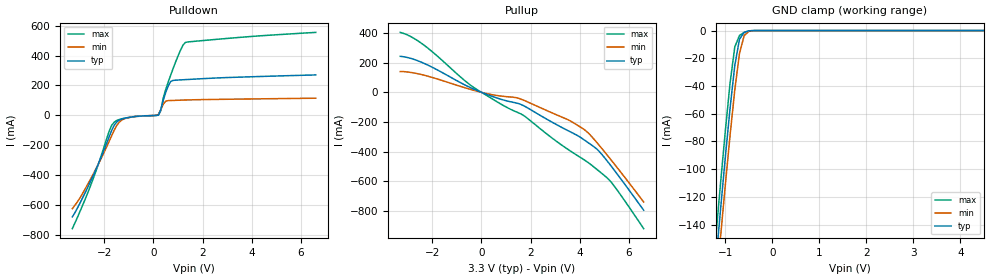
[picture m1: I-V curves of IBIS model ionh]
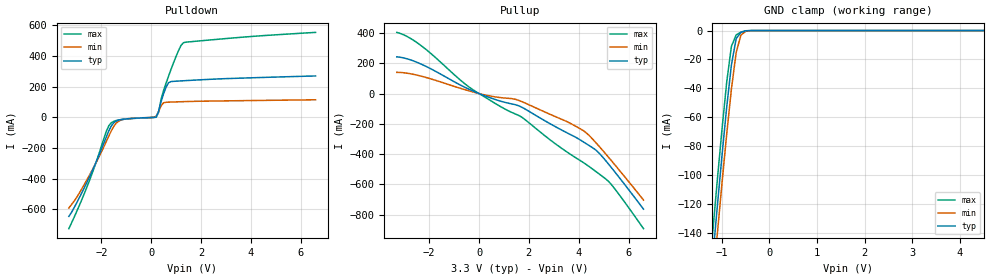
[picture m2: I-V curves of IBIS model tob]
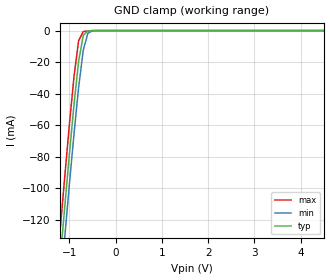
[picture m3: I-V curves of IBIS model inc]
[IBIS Ver]   2.1
[File name]   18512.ibs
[File Rev]   1.0   | from silicon model only
[Date]   97215
[Source]   Silicon-level SPICE model at Texas Instruments (ALEY)
[Notes]
   3.3-V ABT SCAN TEST DEVICES WITH 18-BIT UNIVERSAL BUS TRANSCEIVERS
   Release 1.0) 97215 ALEY - initial release
   includes all available commercial packages:
   DGG=64TSSOP (no-coupling model)
[Disclaimer]
   Property of Texas Instruments Incorporated.  Unauthorized
   reproduction and/or distribution is strictly prohibited.
   This product is protected under copyright law.
   Created 1997, (C) Copyright 1997, Texas Instruments Incorporated.
   All Rights Reserved
   UNLESS THERE IS A SIGNED, WRITTEN AGREEMENT TO THE
   CONTRARY, TEXAS INSTRUMENTS ("TI") IS PROVIDING THE IBIS
   MODELS "AS IS" AND WITHOUT ANY WARRANTY, EXPRESSED OR
   IMPLIED.  TI assumes no liability for:
   1) the accuracy of the IBIS models provided to your
   company;
   2) the proper functioning of these IBIS models in your
   design or for any resulting applications; or
   3) infringement of patents, copyrights or intellectual
   property rights resulting from your use of these IBIS
   models.
   TI provides IBIS Models as a service to our customers.
   You and your company shall not distribute, sell or give
   these models to anyone else without prior written
   permission from TI.
   TI reserves the right to make changes to our products or
   to discontinue any semiconductor product or service
   without notice, and advises our customers to obtain the
   latest version of relevant information to verify, before
   placing orders, that the information being relied on is
   current.
   Please be aware that your receipt and use of the IBIS
   information provided shall serve as acceptance of these
   terms and conditions.  If you do not accept these terms,
   you should return or destroy the IBIS models and any
   other accompanying information immediately.
[Component]   SN74LVT18512DGG
[Manufacturer]  Texas Instruments
[Package]
| 64-pin TSSOP (suffix = DGG)
| variable   typ   min   max
R_pkg   50m   NA   NA
L_pkg   4.0n   NA   NA
C_pkg   0.5p   NA   NA
[Pin]   signal_name   model_name   R_pin   L_pin   C_pin
1   1CLKAB   inc   0.057   5.49n   0.82p
2   1LEAB   inc   0.058   5.10n   0.90p
3   1OEAB#   inu   0.062   4.79n   0.80p
4   1A1   ionh   0.057   4.41n   0.72p
5   1A2   ionh   0.056   4.09n   0.66p
6   GND   GND   0.058   3.86n   0.57p
7   1A3   ionh   0.052   3.54n   0.54p
8   1A4   ionh   0.050   3.34n   0.50p
9   1A5   ionh   0.048   3.12n   0.40p
10   Vcc   POWER   0.046   3.02n   0.39p
11   1A6   ionh   0.049   2.86n   0.35p
12   1A7   ionh   0.046   2.73n   0.34p
13   1A8   ionh   0.043   2.62n   0.33p
14   GND   GND   0.043   2.53n   0.31p
15   1A9   ionh   0.046   2.58n   0.30p
16   2A1   ionh   0.045   2.56n   0.24p
17   2A2   ionh   0.045   2.56n   0.24p
18   2A3   ionh   0.046   2.58n   0.30p
19   GND   GND   0.043   2.53n   0.31p
20   2A4   ionh   0.043   2.62n   0.33p
21   2A5   ionh   0.046   2.73n   0.34p
22   2A6   ionh   0.049   2.86n   0.35p
23   Vcc   POWER   0.046   3.02n   0.39p
24   2A7   ionh   0.048   3.12n   0.40p
25   2A8   ionh   0.050   3.34n   0.50p
26   2A9   ionh   0.052   3.54n   0.54p
27   GND   GND   0.058   3.86n   0.57p
28   2OEAB#   inu   0.056   4.09n   0.66p
29   2LEAB   inc   0.057   4.41n   0.72p
30   2CLKAB   inc   0.062   4.79n   0.80p
31   TDO   tob   0.058   5.10n   0.90p
32   TMS   inu   0.057   5.49n   0.82p
33   TCK   int   0.057   5.49n   0.82p
34   TDI   inu   0.058   5.10n   0.90p
35   2CLKBA   inc   0.062   4.79n   0.80p
36   2LEBA   inc   0.057   4.41n   0.72p
37   2OEBA#   inu   0.056   4.09n   0.66p
38   GND   GND   0.058   3.86n   0.57p
39   2B9   ionh   0.052   3.54n   0.54p
40   2B8   ionh   0.050   3.34n   0.50p
41   2B7   ionh   0.048   3.12n   0.40p
42   Vcc   POWER   0.046   3.02n   0.39p
43   2B6   ionh   0.049   2.86n   0.35p
44   2B5   ionh   0.046   2.73n   0.34p
45   2B4   ionh   0.043   2.62n   0.33p
46   GND   GND   0.043   2.53n   0.31p
47   2B3   ionh   0.046   2.58n   0.30p
48   2B2   ionh   0.045   2.56n   0.24p
49   2B1   ionh   0.045   2.56n   0.24p
50   1B9   ionh   0.046   2.58n   0.30p
51   GND   GND   0.043   2.53n   0.31p
52   1B8   ionh   0.043   2.62n   0.33p
53   1B7   ionh   0.046   2.73n   0.34p
54   1B6   ionh   0.049   2.86n   0.35p
55   Vcc   POWER   0.046   3.02n   0.39p
56   1B5   ionh   0.048   3.12n   0.40p
57   1B4   ionh   0.050   3.34n   0.50p
58   1B3   ionh   0.052   3.54n   0.54p
59   GND   GND   0.058   3.86n   0.57p
60   1B2   ionh   0.056   4.09n   0.66p
61   1B1   ionh   0.057   4.41n   0.72p
62   1OEBA#   inu   0.062   4.79n   0.80p
63   1LEBA   inc   0.058   5.10n   0.90p
64   1CLKBA   inc   0.057   5.49n   0.82p
| Models and submodels in the file (5): ionh (I/O), tob (3-state), inc (Input), int (Input), inu (Input)
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[Model]   ionh
| high-drive I/O buffer (NO bus-hold)
| ibuf.lvta (97212 ALEY)
| tob.lvta  (97212 ALEY)
| pad.lvta  (97212 ALEY)
| Signals   1A1..1A9, 2A1..2A9, 1B1..1B9, 2B1..2B9
Model_type  I/O
Polarity   Non-Inverting
Enable   Active-Low
Vinl = 0.8V
Vinh = 2.0V
| variable   typ   min   max
C_comp   10p   NA   NA
[Temperature Range]   50   100   0
[Voltage range]   3.3   3   3.6
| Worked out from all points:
|   slope of the pulldown table from 0 to 0.495 V, typ, clamps not added: 3.25 ohm
|   slope of the pullup table from 0 to 0.495 V, typ, clamps not added: 16.2 ohm
|   GND clamp passes 1 mA (typ) near -0.57 V on its own axis
|Process range|   weak   strong
[pullup]
|   50C:3.3V:   100C:3V:weak   0C:3.6V:strong
|   Voltage   I(typ)   I(min)   I(max)
-3.3V     242.7mA    140.2mA    404.2mA
-2.8V     225.4mA    132.2mA    369.3mA
-2.3V     192.9mA    114.1mA    313.8mA
-300mV    20.86mA    13.18mA    31.49mA
700mV     -41.88mA   -23.15mA   -70.19mA
1.5V      -75.36mA   -39.76mA   -137.7mA
1.8V      -97.58mA   -58.88mA   -166.1mA
3.6V      -265.1mA   -191.5mA   -393.7mA
4.3V      -334.7mA   -267.1mA   -468.9mA
4.7V      -383.4mA   -339.3mA   -520.3mA
5.2V      -480.9mA   -440.4mA   -590.8mA
6.6V      -795.3mA   -739.8mA   -919.6mA
[pulldown]
|   50C:3.3V:   100C:3V:weak   0C:3.6V:strong
|   Voltage   I(typ)   I(min)   I(max)
-3.3V     -677.8mA   -623.8mA   -757mA
-2.5V     -420.1mA   -407.9mA   -444.4mA
-1.8V     -141.6mA   -172.1mA   -104.6mA
-1.6V     -67.01mA   -100.3mA   -45.5mA
-1.4V     -32.49mA   -46.74mA   -27.91mA
200mV     2.519mA    6.639mA    748.6uA
300mV     39.5mA     39.03mA    32.02mA
500mV     154.3mA    95.61mA    174.8mA
700mV     226.2mA    99.46mA    268.9mA
1.1V      237.3mA    101.8mA    435.7mA
1.3V      239.2mA    102.8mA    487.9mA
6.6V      270.5mA    114.9mA    554.8mA
[gnd_clamp]
|   50C:3.3V:   100C:3V:weak   0C:3.6V:strong
|   Voltage   I(typ)   I(min)   I(max)
-3.3V     -1.549A    -1.512A    -1.612A
-1.2V     -166.3mA   -186.3mA   -147.7mA
-1.1V     -128.1mA   -148mA     -109.1mA
-1V       -90.99mA   -111mA     -72.02mA
-900mV    -55.98mA   -75.55mA   -37.87mA
-800mV    -25.3mA    -42.88mA   -11.86mA
-700mV    -6.208mA   -16.52mA   -3.486mA
-600mV    -1.323mA   -3.594mA   -1.312mA
-500mV    -196.7uA   -581.1uA   -168.7uA
-400mV    -8.354uA   -46.39uA   -1.236uA
6.6V      9.206nA    10.07nA    9.034nA
[ramp]
| variable   typ   min   max
dV/dt_r   1.5082E+00/4.7934E-10  1.1408E+00/1.4421E-09  1.7780E+00/2.2208E-10
dV/dt_f   1.7910E+00/8.5440E-10  1.6176E+00/2.2829E-09  1.9765E+00/4.0622E-10
[Model]   tob
| three-state output buffer
| tob.lvta (97212 ALEY)
| pad.lvta (97212 ALEY)
| Signals   TDO
Model_type  3-state
Polarity   Non-Inverting
Enable   Active-Low
| variable   typ   min   max
C_comp   8p   NA   NA
[Temperature Range]   50   100   0
[Voltage range]   3.3   3   3.6
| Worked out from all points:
|   slope of the pulldown table from 0 to 0.495 V, typ, clamps not added: 3.25 ohm
|   slope of the pullup table from 0 to 0.495 V, typ, clamps not added: 16.2 ohm
|   GND clamp passes 1 mA (typ) near -0.58 V on its own axis
|Process range|   weak   strong
[pullup]
|   50C:3.3V:   100C:3V:weak   0C:3.6V:strong
|   Voltage   I(typ)   I(min)   I(max)
-3.3V     242.7mA    140.2mA    404.2mA
-2.8V     225.4mA    132.2mA    369.3mA
-2.3V     192.9mA    114.1mA    313.8mA
-300mV    20.86mA    13.18mA    31.49mA
700mV     -41.88mA   -23.15mA   -70.19mA
1.5V      -75.36mA   -39.76mA   -137.7mA
1.8V      -97.58mA   -58.87mA   -166.1mA
3.6V      -265.1mA   -191mA     -393.7mA
4.3V      -331mA     -259mA     -468.4mA
4.7V      -375mA     -326.3mA   -516.3mA
5.2V      -466.4mA   -421.4mA   -580.8mA
6.6V      -763.6mA   -703.5mA   -892.5mA
[pulldown]
|   50C:3.3V:   100C:3V:weak   0C:3.6V:strong
|   Voltage   I(typ)   I(min)   I(max)
-3.3V     -646.1mA   -591.2mA   -726.1mA
-2.5V     -398.2mA   -385.2mA   -423.3mA
-1.8V     -128.3mA   -158mA     -92.21mA
-1.6V     -56.18mA   -88.6mA    -35.51mA
-1.4V     -24.07mA   -37.43mA   -20.33mA
200mV     2.519mA    6.639mA    748.6uA
300mV     39.5mA     39.03mA    32.02mA
500mV     154.3mA    95.61mA    174.8mA
700mV     226.2mA    99.46mA    268.9mA
1.1V      237.3mA    101.8mA    435.7mA
1.3V      239.2mA    102.8mA    487.9mA
6.6V      270.5mA    114.9mA    554.8mA
[gnd_clamp]
|   50C:3.3V:   100C:3V:weak   0C:3.6V:strong
|   Voltage   I(typ)   I(min)   I(max)
-3.3V     -1.517A    -1.479A    -1.581A
-1.2V     -160.3mA   -179.4mA   -142.5mA
-1.1V     -123.2mA   -142.2mA   -105mA
-1V       -87.28mA   -106.4mA   -69.11mA
-900mV    -53.39mA   -72.1mA    -36.02mA
-800mV    -23.77mA   -40.53mA   -10.91mA
-700mV    -5.596mA   -15.18mA   -3.038mA
-600mV    -1.236mA   -3.105mA   -1.085mA
-500mV    -194.2uA   -518.2uA   -118.5uA
-400mV    -8.285uA   -43.13uA   -1.218uA
6.6V      7.886nA    8.661nA    7.714nA
[ramp]
| variable   typ   min   max
dV/dt_r   1.5081E+00/4.7366E-10  1.1387E+00/1.4512E-09  1.7781E+00/2.1597E-10
dV/dt_f   1.7910E+00/8.4858E-10  1.6182E+00/2.2837E-09  1.9768E+00/4.0623E-10
[Model]   inc
| high-impedance input buffer
| iclk.lvta (97212 ALEY)
| pad.lvta  (97212 ALEY)
| Signals   CLK, LE
Model_type  Input
Polarity   Non-Inverting
Vinl = 0.8V
Vinh = 2.0V
| variable   typ   min   max
C_comp   4p   NA   NA
[Temperature Range]   50   100   0
[Voltage range]   3.3   3   3.6
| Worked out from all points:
|   GND clamp passes 1 mA (typ) near -0.63 V on its own axis
|Process range|   weak   strong
[gnd_clamp]
|   50C:3.3V:   100C:3V:weak   0C:3.6V:strong
|   Voltage   I(typ)   I(min)   I(max)
-3.3V     -902.8mA   -920.5mA   -885.5mA
-1.2V     -145.7mA   -165.1mA   -126.6mA
-1.1V     -111.6mA   -131mA     -92.49mA
-1V       -78.36mA   -97.58mA   -59.49mA
-900mV    -46.84mA   -65.49mA   -29.02mA
-800mV    -19.33mA   -35.9mA    -6.331mA
-700mV    -3.025mA   -12.3mA    -602.9uA
-600mV    -177.8uA   -1.693mA   -229.1uA
-500mV    -5.2uA     -126.4uA   -50.31uA
6.6V      1.98nA     2.082nA    1.98nA
